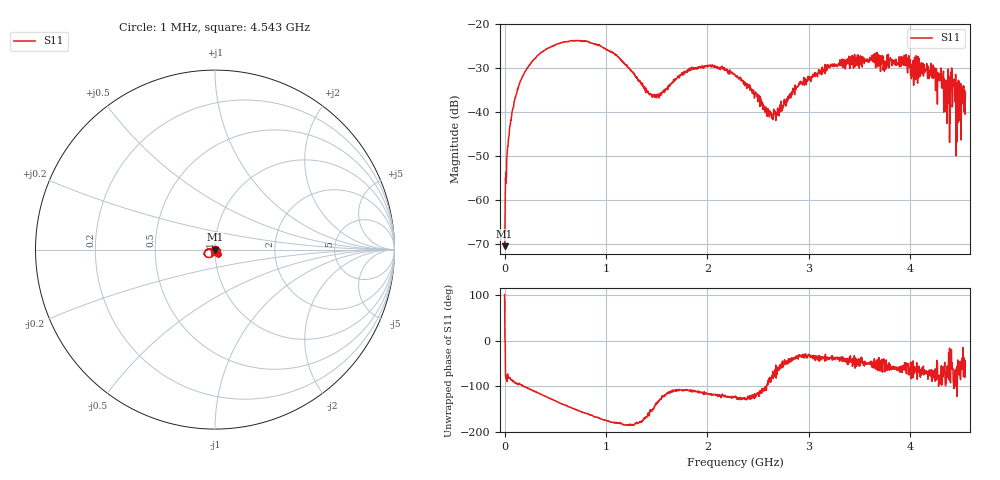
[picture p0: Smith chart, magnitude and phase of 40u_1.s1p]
# HZ S RI R 50
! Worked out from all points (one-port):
!   1515 points, 1 MHz to 4.543 GHz, reference 50 ohm
!   lowest |S11| = -70.5 dB at 1 MHz (marker M1), VSWR 1.00, Z = 50 + j0.0294 ohm
!   |S11| at or under -10 dB: start of sweep to end of sweep
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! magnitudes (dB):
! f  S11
! 1 MHz  -70.5
! 28 MHz  -48.8
! 43 MHz  -45.6
! 82 MHz  -39.1
! 142 MHz  -33.9
! 319 MHz  -27.3
! 571 MHz  -24.1
! 814 MHz  -23.9
! 1.138 GHz  -27.8
! 1.468 GHz  -36.4
! 1.705 GHz  -32.1
! 2.026 GHz  -29.4
! 2.272 GHz  -31.4
! 2.629 GHz  -40.1
! 2.695 GHz  -40.7
! 2.842 GHz  -34.7
! 3.199 GHz  -29.9
! 3.409 GHz  -29.1
! 3.976 GHz  -30.1
! 4.012 GHz  -32.4
! 4.144 GHz  -30.6
! 4.306 GHz  -32.8
! 4.366 GHz  -37.2
! 4.39 GHz  -32.8
! 4.408 GHz  -29.9
! 4.417 GHz  -38.0
! 4.471 GHz  -42.4
! 4.543 GHz  -35.7
